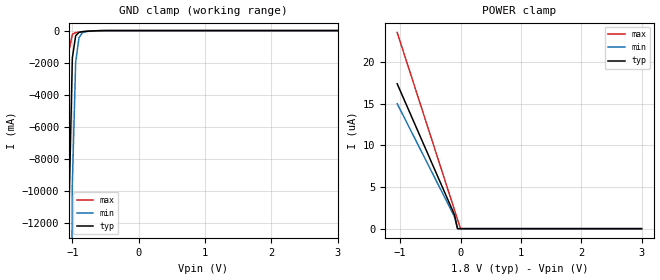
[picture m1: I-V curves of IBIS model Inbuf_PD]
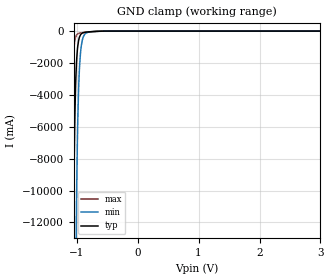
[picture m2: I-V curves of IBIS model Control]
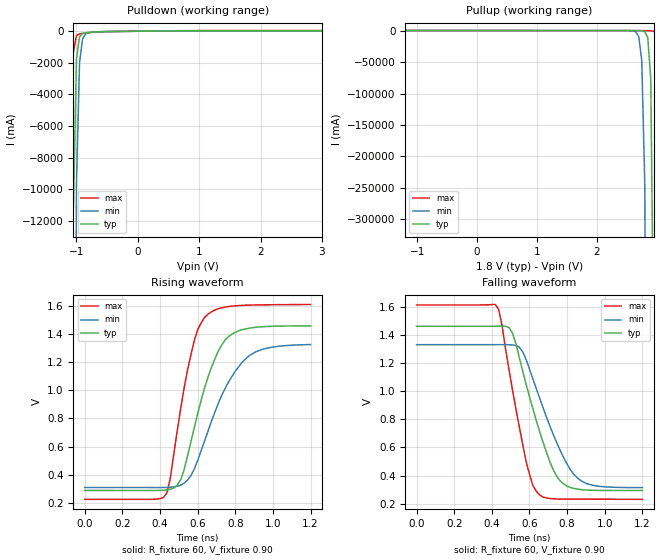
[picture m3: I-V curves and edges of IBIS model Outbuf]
|   This file is an IBIS representation of the   |
|   CDCU877B provided by Texas Instruments   |
| This file contains preliminary package information for the following types:
|  uBGA 52-ball (GQL) package as [Component] cdcu877bgql
|   MLF 40-pin  (RTB) package as [Component] cdcu877brtb
|=================== Header Section -------------------------------------------|
[IBIS Ver]   3.2
[File Name]   cdcu877b.ibs
[File Rev]   1.0
[Date]   18 Mai 2005 | Last modified
|   18 Mai 2005 | Created
[Source]   This file originated at Texas Instruments
|   this file was generated based on simulation results of TI-Spice
|REVISON LOG:01 initial version
[Notes]
[Disclaimer]
(C) Copyright Texas Instruments Incorporated 2003
   All rights reserved
  Texas Instruments Incorporated hereby grants the user of this IBIS
model a non-exclusive, nontransferable license to use this IBIS model
under the following terms.  Before using this IBIS model, the user
should read this license.  If the user does not accept these terms,
the IBIS model should be returned to Texas Instruments within 30 days.
  The user is granted this license only to use the IBIS model and
is not granted rights to sell, load, rent, lease or license the IBIS
model in whole or in part, or in modified form to anyone other than
user.  User may modify the IBIS model to suit its specific applications
but rights to derivative works and such modifications shall belong to
Texas Instruments.
  This IBIS model is provided on an "AS IS" basis and Texas Instruments
makes absolutely no warranty with respect to the information contained
herein.  TEXAS INSTRUMENTS DISCLAIMS AND CUSTOMER WAIVES ALL WARRANTIES,
EXPRESS OR IMPLIED, INCLUDING WARRANTIES OF MERCHANTABILITY OR FITNESS
FOR A PARTICULAR PURPOSE. The entire risk as to quality and performance
is with the Customer. ACCORDINGLY, IN NO EVENT SHALL THE COMPANY BE LIABLE
FOR ANY DAMAGES, WHETHER IN CONTRACT OR TORT,INCLUDING ANY LOST PROFITS
OR OTHER INCIDENTAL, CONSEQUENTIAL, EXEMPLARY, OR PUNITIVE DAMAGES ARISING
OUT OF THE USE OR APPLICATION OF THE IBIS model provided in this package.
Further, Texas Instruments reserves the right to discontinue or make changes
without notice to any product herein to improve reliability, function, or
design. Texas Instruments does not convey any license under patent rights
or any other intellectual property rights, including those of third parties.
Contact Texas Instruments at ATTN: HPA-High Speed Communication & Control, HSCC
[Copyright]   Copyright (C)2003 Texas Instruments, All Rights Reserved
|------------------- End of Header Section ====================================|
|=================== Component Section ----------------------------------------|
| Component CDCU877BGQL, 52-ball, uBGA
[Component]   CDCU877BGQL   |Name of Device
[Manufacturer]  Texas Instruments
[Package]
|   typ   min   max
R_pkg   0.12Ohm   0.05Ohm   0.30Ohm
L_pkg   2.38nH   1.13nH   5.66nH
C_pkg   0.11pF   0.04pF   0.47pF
|pinout for uBGA package
[Pin] signal_name  model_name   R_pin   L_pin   C_pin
 D2   VDDQ   POWER   0.114Ohm   2.881nH   0.188pF
 C1   Y2-   Outbuf   0.114Ohm   2.285nH   0.085pF
 D1   Y2   Outbuf   0.094Ohm   1.872nH   0.079pF
 C2   GND   GND   0.080Ohm   2.098nH   0.257pF
 E1   CK   Inbuf_PD   0.087Ohm   1.754nH   0.074pF
 F1   CK-   Inbuf_PD   0.088Ohm   1.761nH   0.078pF
 F2   VDDQ   POWER   0.112Ohm   2.382nH   0.127pF
 G1   AGND   GND   0.051Ohm   1.129nH   0.079pF
 H1   AVDD   POWER   0.058Ohm   1.250nH   0.088pF
 G2   VDDQ   POWER   0.102Ohm   2.270nH   0.164pF
 H2   GND   GND   0.162Ohm   3.098nH   0.120pF
 J1   Y3   Outbuf   0.134Ohm   2.519nH   0.052pF
 K1   Y3-   Outbuf   0.134Ohm   2.519nH   0.052pF
 J2   GND   GND   0.122Ohm   2.311nH   0.053pF
 K2   Y4-   Outbuf   0.124Ohm   2.347nH   0.060pF
 K3   Y4   Outbuf   0.122Ohm   2.307nH   0.060pF
 G3   VDDQ   POWER   0.163Ohm   3.559nH   0.133pF
 K4   Y9   Outbuf   0.123Ohm   2.322nH   0.060pF
 K5   Y9-   Outbuf   0.126Ohm   2.381nH   0.060pF
 J5   GND   GND   0.071Ohm   1.447nH   0.220pF
 K6   Y8-   Outbuf   0.140Ohm   2.627nH   0.051pF
 J6   Y8   Outbuf   0.136Ohm   2.481nH   0.044pF
 G4   VDDQ   POWER   0.165Ohm   2.258nH   0.300pF
 D5   OS   Control   0.300Ohm   5.663nH   0.467pF
 F5   OE   Control   0.122Ohm   2.504nH   0.346pF
 H6   FBOUT   Outbuf   0.110Ohm   2.156nH   0.104pF
 G6   FBOUT-   Outbuf   0.100Ohm   1.961nH   0.074pF
 H5   GND   GND   0.153Ohm   3.024nH   0.173pF
 F6   FBIN-   Inbuf   0.089Ohm   1.779nH   0.075pF
 E6   FBIN   Inbuf   0.088Ohm   1.784nH   0.078pF
 E5   VDDQ   POWER   0.108Ohm   2.318nH   0.122pF
 D6   Y7   Outbuf   0.095Ohm   1.887nH   0.079pF
 C6   Y7-   Outbuf   0.106Ohm   2.129nH   0.083pF
 C5   GND   GND   0.088Ohm   1.872nH   0.139pF
 D4   VDDQ   POWER   0.134Ohm   3.050nH   0.200pF
 B6   Y6-   Outbuf   0.134Ohm   2.524nH   0.053pF
 A6   Y6   Outbuf   0.136Ohm   2.555nH   0.052pF
 B5   GND   GND   0.123Ohm   2.340nH   0.053pF
 A5   Y5   Outbuf   0.125Ohm   2.367nH   0.060pF
 A4   Y5-   Outbuf   0.123Ohm   2.322nH   0.061pF
 D3   VDDQ   POWER   0.159Ohm   3.476nH   0.128pF
 A3   Y0-   Outbuf   0.122Ohm   2.306nH   0.061pF
 A2   Y0   Outbuf   0.124Ohm   2.345nH   0.061pF
 B2   GND   GND   0.122Ohm   2.311nH   0.053pF
 A1   Y1   Outbuf   0.131Ohm   2.474nH   0.052pF
 B1   Y1-   Outbuf   0.129Ohm   2.444nH   0.052pF
[Diff_Pin]  inv_pin  vdiff   tdelay_typ  tdelay_min  tdelay_max
| The '+' pin is   Diff_pin,   the '-' pin is the   Inv_pin
| Receiver Pins  |  Receiver Vth = +/-300mV (DC, AC=0.6V)
E1   F1   0.3V   0ns   0ns   0ns   | CK  / CK-
E6   F6   0.3V   0ns   0ns   0ns   | FBIN/ FBIN-
| Driver Pins   |  Rload = xx ohm at xx termination
D1   C1   NA   0ns   0ns   0ns   | Y2 / Y2-
A1   B1   NA   0ns   0ns   0ns   | Y1 / Y1-
J1   K1   NA   0ns   0ns   0ns   | Y3 / Y3-
A2   A3   NA   0ns   0ns   0ns   | Y0 / Y0-
A5   A4   NA   0ns   0ns   0ns   | Y5 / Y5-
A6   B6   NA   0ns   0ns   0ns   | Y6 / Y6-
D6   C6   NA   0ns   0ns   0ns   | Y7 / Y7-
J6   K6   NA   0ns   0ns   0ns   | Y8 / Y8-
K4   K5   NA   0ns   0ns   0ns   | Y9 / Y9-
K3   K2   NA   0ns   0ns   0ns   | Y4 / Y4-
H6   G6   NA   0ns   0ns   0ns   | FBOUT / FBOUT-
| Component CDCU877BRTB 40-pin MLF
[Component]   CDCU877BRTB   |Name of Device
[Manufacturer]  Texas Instruments
[Package]
|   typ   min   max
R_pkg   0.12Ohm   0.06Ohm   0.15Ohm
L_pkg   1.17nH   0.59nH   1.50nH
C_pkg   0.07pF   0.03pF   0.11pF
|pinning for MLF40 package
[Pin] signal_name  model_name   R_pin   L_pin   C_pin
  1   VDDQ   POWER   0.071Ohm   0.706nH   0.095pF
  2   Y2-   Outbuf   0.133Ohm   1.319nH   0.080pF
  3   Y2   Outbuf   0.124Ohm   1.229nH   0.111pF
  4   CK   Inbuf_PD   0.121Ohm   1.194nH   0.099pF
  5   CK-   Inbuf_PD   0.117Ohm   1.156nH   0.060pF
  6   VDDQ   POWER   0.117Ohm   1.157nH   0.070pF
  7   AGND   GND   0.060Ohm   0.592nH   0.071pF
  8   AVDD   POWER   0.062Ohm   0.609nH   0.072pF
  9   VDDQ   POWER   0.064Ohm   0.632nH   0.074pF
 10   GND   GND   0.143Ohm   1.419nH   0.078pF
 11   Y3   Outbuf   0.146Ohm   1.442nH   0.071pF
 12   Y3-   Outbuf   0.133Ohm   1.321nH   0.048pF
 13   Y4-   Outbuf   0.128Ohm   1.267nH   0.085pF
 14   Y4   Outbuf   0.121Ohm   1.195nH   0.063pF
 15   VDDQ   POWER   0.117Ohm   1.157nH   0.056pF
 16   Y9   Outbuf   0.117Ohm   1.156nH   0.055pF
 17   Y9-   Outbuf   0.121Ohm   1.195nH   0.056pF
 18   Y8-   Outbuf   0.125Ohm   1.233nH   0.057pF
 19   Y8   Outbuf   0.134Ohm   1.325nH   0.054pF
 20   VDDQ   POWER   0.071Ohm   0.700nH   0.076pF
 21   OS   Control   0.145Ohm   1.439nH   0.077pF
 22   OE   Control   0.133Ohm   1.318nH   0.084pF
 23   VDDQ   POWER   0.124Ohm   1.229nH   0.073pF
 24   FBOUT   Outbuf   0.118Ohm   1.173nH   0.061pF
 25   FBOUT-   Outbuf   0.116Ohm   1.152nH   0.073pF
 26   FBIN-   Inbuf   0.117Ohm   1.157nH   0.070pF
 27   FBIN   Inbuf   0.121Ohm   1.196nH   0.074pF
 28   VDDQ   POWER   0.128Ohm   1.272nH   0.075pF
 29   Y7   Outbuf   0.139Ohm   1.375nH   0.081pF
 30   Y7-   Outbuf   0.151Ohm   1.500nH   0.041pF
 31   VDDQ   POWER   0.071Ohm   0.705nH   0.081pF
 32   Y6-   Outbuf   0.133Ohm   1.316nH   0.097pF
 33   Y6   Outbuf   0.124Ohm   1.227nH   0.060pF
 34   Y5   Outbuf   0.120Ohm   1.192nH   0.049pF
 35   Y5-   Outbuf   0.117Ohm   1.156nH   0.054pF
 36   VDDQ   POWER   0.117Ohm   1.158nH   0.049pF
 37   Y0-   Outbuf   0.121Ohm   1.198nH   0.033pF
 38   Y0   Outbuf   0.129Ohm   1.274nH   0.025pF
 39   Y1   Outbuf   0.134Ohm   1.330nH   0.101pF
 40   Y1-   Outbuf   0.146Ohm   1.447nH   0.084pF
Pad   GND   GND   0.007Ohm   0.064nH   0.355pF
[Diff_Pin]  inv_pin  vdiff   tdelay_typ  tdelay_min  tdelay_max
| The '+' pin is   Diff_pin,   the '-' pin is the   Inv_pin
| Receiver Pins  |  Receiver Vth = +/-300mV (DC, AC=0.6V)
4   5   0.3V   0ns   0ns   0ns   | CK  / CK-
27   26   0.3V   0ns   0ns   0ns   | FBIN/ FBIN-
| Driver Pins   |  Rload = xx ohm at xx termination
3   2   NA   0ns   0ns   0ns   | Y2 / Y2-
11   12   NA   0ns   0ns   0ns   | Y3 / Y3-
14   13   NA   0ns   0ns   0ns   | Y4 / Y4-
16   17   NA   0ns   0ns   0ns   | Y9 / Y9-
19   18   NA   0ns   0ns   0ns   | Y8 / Y8-
24   25   NA   0ns   0ns   0ns   | FBOUT / FBOUT-
29   30   NA   0ns   0ns   0ns   | Y7 / Y7-
33   32   NA   0ns   0ns   0ns   | Y6 / Y6-
34   35   NA   0ns   0ns   0ns   | Y5 / Y5-
38   37   NA   0ns   0ns   0ns   | Y0 / Y0-
39   40   NA   0ns   0ns   0ns   | Y1 / Y1-
|------------------- End of Component Section ==============================
| Models and submodels in the file (4): Inbuf_PD (Input), Control (Input), Inbuf (Input), Outbuf (Output)
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|=================== Models Section ----------------------------------------
|   Model   Inbuf_PD
[Model]   Inbuf_PD
Model_type   Input
|Signals   CK, CK-
Polarity   Non-Inverting
Vinl   =   0.665
Vinh   =   1.105
|Variable   typ   min   max
C_comp   1.862e-12   1.846e-12   1.888e-12
|Variable   typ   min   max
[Voltage range]   1.8   1.7   1.9
|Variable   typ   min   max
[Temperature range]  27   85   -40
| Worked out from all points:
|   GND clamp passes 1 mA (typ) near -0.50 V on its own axis
[GND_clamp]
|Volts   typ   min   max
-1.05V    -11.13A    -48.06A    -1.266A
-1V       -1.703A    -9.594A    -232.9mA
-950mV    -324.9mA   -1.97A     -126.8mA
-900mV    -111.4mA   -449.6mA   -98.18mA
-850mV    -67.16mA   -137.4mA   -76.69mA
-750mV    -34.25mA   -40.96mA   -38.72mA
-500mV    -910.7uA   -2.133mA   -368.9uA
3V        29.81uA    24.29uA    42.62uA
[POWER_clamp]
|Volts   typ   min   max
-1.05V    17.39uA    15uA       23.55uA
-100mV    1.656uA    1.429uA    2.243uA
-50mV     0A         0A         1.121uA
0V        0A         0A         0A
3V        0A         0A         0A
|   Model   Control
[Model]   Control
Model_type   Input
|Signals   OS, OE
Polarity   Non-Inverting
Vinl   =   0.665
Vinh   =   1.105
|Variable   typ   min   max
C_comp   1.296e-12   1.287e-12   1.315e-12
|Variable   typ   min   max
[Voltage range]   1.8   1.7   1.9
|Variable   typ   min   max
[Temperature range]  27   85   -40
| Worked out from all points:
|   GND clamp passes 1 mA (typ) near -0.50 V on its own axis
[GND_clamp]
|Volts   typ   min   max
-1.05V    -11.12A    -48.06A    -1.264A
-1.045V   -9.19A     -40.89A    -1.019A
-1.03V    -5.196A    -25.19A    -560.2mA
-1.015V   -2.957A    -15.53A    -339.2mA
-1.005V   -2.043A    -11.26A    -259.1mA
-1V       -1.702A    -9.593A    -231.1mA
-985mV    -996.2mA   -5.937A    -176.3mA
-970mV    -599mA     -3.686A    -146.9mA
-955mV    -374.5mA   -2.301A    -129.6mA
-910mV    -129.3mA   -593.6mA   -101.5mA
-855mV    -68.87mA   -150.9mA   -77.71mA
3V        0A         0A         0A
[POWER_clamp]
|Volts   typ   min   max
-1.05V    0A         0A         0A
0V        0A         0A         0A
3V        0A         0A         0A
|   Model   Outbuf
[Model]   Outbuf
Model_type   Output
Polarity   Non-Inverting
Vmeas  =   0.90
Cref   =   10pF
Rref   =   60
Vref   =   0.90
|Variable   typ   min   max
C_comp   1.941e-12   1.868e-12   1.950e-12
[Model Spec]
|  subparameter   typ   min   max
Vmeas   0.905V   0.869V   0.970V
|Variable   typ   min   max
[Voltage range]   1.8   1.7   1.9
|Variable   typ   min   max
[Temperature range]  27   85   -40
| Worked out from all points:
|   slope of the pulldown table from 0 to 0.27 V, typ, clamps not added: 28.3 ohm
|   slope of the pullup table from 0 to 0.27 V, typ, clamps not added: 35.7 ohm
|   rising waveform, R_fixture 60, V_fixture 0.90: 20-80 % time 147ps typ, 190ps min, 110ps max; typ from 0.289 V to 1.46 V
|   falling waveform, R_fixture 60, V_fixture 0.90: 20-80 % time 153ps typ, 178ps min, 112ps max; typ from 1.46 V to 0.293 V
[Pulldown]
|Voltage   I(typ)   I(min)   I(max)
-1.05V    -11.16A    -48.09A    -1.312A
-1V       -1.735A    -9.621A    -277.5mA
-950mV    -355.5mA   -1.996A    -170mA
-900mV    -140.9mA   -474.4mA   -139.8mA
-850mV    -95.37mA   -161.2mA   -116.7mA
-750mV    -59.92mA   -62.54mA   -75.41mA
-450mV    -16.77mA   -14.69mA   -23.89mA
3V        33.58mA    29.57mA    47.36mA
[Pullup]
|Voltage   I(typ)   I(min)   I(max)
-1.2V     36.27mA    30.7mA     47.37mA
2.5V      -52.54mA   -84.92mA   -50.46mA
2.65V     -96.13mA   -1.989A    -83.74mA
2.7V      -140mA     -9.613A    -101.4mA
2.75V     -353.1mA   -48.08A    -120.7mA
2.8V      -1.731A    -242.4A    -141.6mA
2.85V     -11.15A    -1.224kA   -169.7mA
2.9V      -76.17A    -6.187kA   -275.2mA
2.95V     -525.5A    -31.27kA   -1.308A
[Ramp]
|Variable   typ   min   max
dV/dt_r  0.8635/1.804e-10   0.7468/2.306e-10   0.9694/1.299e-10
dV/dt_f  0.9054/2.031e-10   0.8158/2.417e-10   1.0116/1.399e-10
R_load  =  152  | 120ohms + 1x channel impedance (HIGH+LOW)/2= 31.85ohms
| R_load = differential termination 120ohm channel to channel,
|   or single-ended with Rload to common mode voltage.
[Rising Waveform]
R_fixture   =   60
V_fixture   =   0.90
V_fixture_min   =   0.85
V_fixture_max   =   0.95
C_fixture   =   0.00
|Time   V(typ)   V(min)   V(max)
0s        289mV      310.3mV    226.3mV
436.4ps   293mV      310.7mV    271.2mV
454.5ps   297.6mV    311.9mV    374.6mV
509.1ps   362.6mV    326.4mV    863.2mV
563.6ps   631mV      392.9mV    1.248V
600ps     833.8mV    502.2mV    1.43V
654.5ps   1.091V     708.6mV    1.54V
745.5ps   1.356V     1.012V     1.591V
872.7ps   1.441V     1.245V     1.605V
1.2ns     1.457V     1.325V     1.609V
[Falling Waveform]
R_fixture   =   60
V_fixture   =   0.90
V_fixture_min   =   0.85
V_fixture_max   =   0.95
C_fixture   =   0.00
|Time   V(typ)   V(min)   V(max)
0s        1.462V     1.332V     1.614V
436.4ps   1.463V     1.332V     1.583V
509.1ps   1.416V     1.329V     1.014V
545.5ps   1.241V     1.315V     749.4mV
581.8ps   1.05V      1.227V     501.1mV
618.2ps   874.4mV    1.087V     328.7mV
654.5ps   710.1mV    948.3mV    261.2mV
745.5ps   392.8mV    631.4mV    232.7mV
854.5ps   303.1mV    382mV      231.6mV
1.2ns     293.4mV    313.7mV    230.4mV
